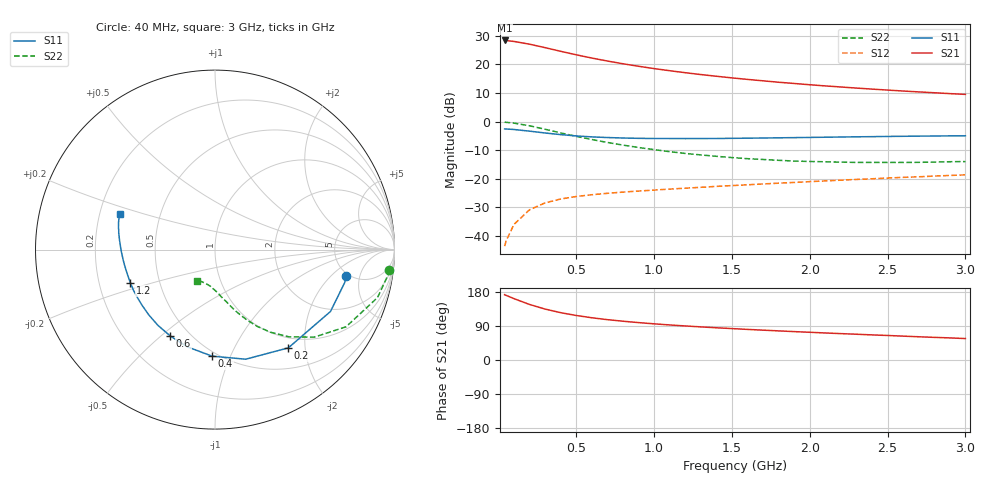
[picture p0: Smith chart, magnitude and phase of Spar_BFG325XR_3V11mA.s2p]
! Filename: 311BFG325XR.s2p
! Title: BFG325XR,RN20042071,Lot:TT3899C,B:Y13641,Sl.:1
! Bias: VCE=2.999V; IC=10.90mA;
! Company: NXP Semiconductors NL
! User: Q&R DSC-N
! Measure time: 29 Mar 2004 / 13:39:54
#  MHz  S  MA  R 50
! Freq  S11  S21  S12  S22  :
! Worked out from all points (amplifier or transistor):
!   32 points, 40 MHz to 3 GHz, reference 50 ohm
!   highest |S21| = 28.4 dB at 40 MHz (marker M1)
!   |S21| within 3 dB of that: start of sweep to 338 MHz
!   unconditionally stable (mu >= 1): 2.078 GHz to end of sweep
!   at 400 MHz: K = 0.35, MSG = 25.8 dB, |S12| = -27.0 dB
!   at 1.5 GHz: K = 0.90, MSG = 18.8 dB, |S12| = -22.3 dB
!   at 3 GHz: K = 1.05, MAG = 12.7 dB, |S12| = -18.6 dB
!   S11 on the Smith chart (normalised r, x): 40 MHz: 4.72, -3.17; 200 MHz: 0.82, -1.69; 400 MHz: 0.47, -0.86; 600 MHz: 0.39, -0.54; 1.2 GHz: 0.34, -0.17; 3 GHz: 0.28, +0.16
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40  0.7471 -11.4  26.29 172.4  0.006664 84.1  0.9784 -6.6
50  0.7456 -14.3  26.14 170.6  0.008304 82.7  0.9745 -8.3
100  0.7301 -28.2  25.28 161.9  0.01599 76.3  0.9442 -16.4
200  0.6831 -53.3  22.64 146.6  0.02882 65.2  0.8476 -30.5
300  0.6342 -74.4  19.69 134.4  0.03805 57.2  0.7373 -41.4
400  0.594 -91.5  16.99 124.9  0.04448 51.8  0.6369 -49.7
500  0.5635 -105.7  14.76 117.5  0.04921 48.4  0.5542 -56.1
600  0.5421 -117.4  12.96 111.5  0.05285 46.2  0.4877 -61.2
700  0.5283 -127.1  11.49 106.5  0.05591 44.9  0.4336 -65.3
800  0.5182 -135.2  10.29 102.3  0.05876 44.3  0.3897 -68.9
900  0.5115 -142.3  9.308 98.7  0.06128 44.0  0.3541 -72.0
1000  0.5082 -148.5  8.48 95.4  0.06376 44.0  0.3247 -74.8
1100  0.5076 -153.8  7.781 92.5  0.06632 44.1  0.2991 -77.5
1200  0.5061 -158.6  7.18 89.9  0.06874 44.3  0.2785 -80.3
1300  0.5069 -162.9  6.668 87.4  0.07124 44.6  0.2623 -82.9
1400  0.5085 -166.8  6.227 85.0  0.0739 44.9  0.2482 -85.2
1600  0.5146 -173.4  5.486 80.7  0.07882 45.6  0.2256 -90.4
1800  0.5224 -179.0  4.892 76.8  0.0841 46.3  0.2111 -95.0
2100  0.535 174.1  4.217 71.3  0.09215 46.9  0.199 -102.2
2300  0.5441 170.3  3.866 68.0  0.09785 47.2  0.1939 -106.5
2600  0.5552 165.4  3.433 63.0  0.1063 47.5  0.1937 -112.7
3000  0.5668 159.8  2.999 56.6  0.1176 47.0  0.201 -119.8
